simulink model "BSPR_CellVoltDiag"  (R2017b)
settings: Solver=FixedStepDiscrete  StartTime=0.0  StopTime=10.0  FixedStep=0.02  RelTol=1e-3  EnableMultiTasking=on
undefined symbols (not defined in the file): bin2dec, BSPR_bCellVoltAlrmDiag_C, BSPR_CellNplDetVoltThres_C, BSPR_cntCellAvlNum_C, BSPR_cntCellVltRngEnvtCsdr_CW, BSPR_cntCellVoltNplDiag_CW, BSPR_cntCellVoltRngDiag_CW, BSPR_cntModuAvlNum_C, BSPR_cntUCellNplErrThres_C, BSPR_cntUCellNplOkThres_C, BSPR_cntVoltCellMeanSwt_CW, BSPR_cofCurrFltCellRng_C, BSPR_iCellVoltRngCurrHi_C, BSPR_iCellVoltRngCurrLo_C, BSPR_iCurrHopFltDiff_C, BSPR_tBattTempCellVoltRngHi_C, BSPR_tBattTempCellVoltRngLo_C, BSPR_tEnvTCellVoltRngHi_C, BSPR_tEnvTCellVoltRnglo_C, BSPR_tiCellVoltAlrm_C, BSPR_tiCellVoltDiagTask_C, BSPR_tiCellVoltFault_C, BSPR_tiCellVoltFusf_C, BSPR_tiCellVoltWarn_C, BSPR_tiUCellNplErrThres_C, BSPR_tiUCellNplOkThres_C, BSPR_uCellVoltNplDiag_CUR, BSPR_uCellVoltNplDiag_CUR_X, BSPR_uCellVoltRng_CUR_X, BSPR_uCellVoltRng_CUR_Y, BSPR_uCellVoltRngHiFault_CUR, BSPR_uCellVoltRngHiFusf_CUR, BSPR_uCellVoltRngHiWarnAlrm_CUR, BSPR_uCellVoltRngLoFault_CUR, BSPR_uCellVoltRngLoFusf_CUR, BSPR_uCellVoltRngLoWarnAlrm_CUR
libraries: simulink x68, AIWAYS_Powertrain_BMS_lib x9
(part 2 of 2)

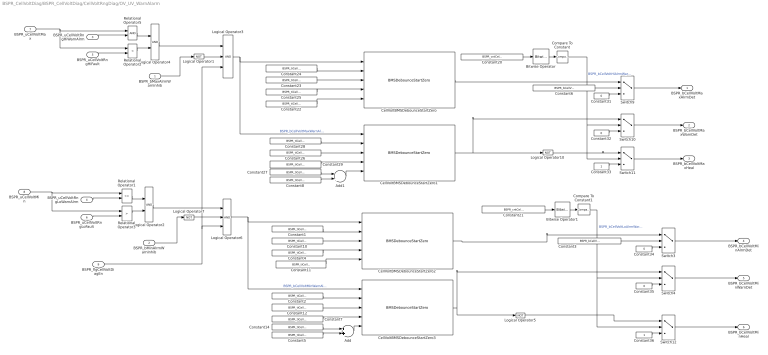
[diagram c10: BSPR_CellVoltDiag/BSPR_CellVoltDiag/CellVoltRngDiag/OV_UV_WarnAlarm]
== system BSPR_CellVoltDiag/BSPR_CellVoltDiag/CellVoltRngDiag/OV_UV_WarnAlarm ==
  BSPR_bMaxAlrmWarnInhib : Inport
  BSPR_bMinAlrmWarnInhib : Inport  Port=2
  BSPR_uCellVoltRngHiWarnAlrm : Inport  Port=3
  BSPR_uCellVoltRngLoWarnAlrm : Inport  Port=4
  BSPR_uCellVoltRngHiFault : Inport  Port=5
  BSPR_uCellVoltRngLoFault : Inport  Port=6
  BSPR_uCellVoltMax : Inport  Port=7
  BSPR_uCellVoltMin : Inport  Port=8
  BSPR_flgCellVoltDiagEn : Inport  Port=9
  Add : Sum
  Add1 : Sum
  Bitwise Operator : simulink/Logic and Bit Operations/Bitwise Operator  logicop=AND  UseBitMask=on  BitMask=bin2dec('00000001')  BitMaskRealWorld=Stored Integer
  Bitwise Operator1 : simulink/Logic and Bit Operations/Bitwise Operator  logicop=AND  UseBitMask=on  BitMask=bin2dec('00000010')  BitMaskRealWorld=Stored Integer
  CellVoltBMSDebounceStartZero{,1..3} (4 alike) : AIWAYS_Powertrain_BMS_lib/Debounce & Delay/BMSDebounceStartZero
  Compare To Constant : simulink/Logic and Bit Operations/Compare To Constant  relop===  const=1  OutDataTypeStr=boolean
  Compare To Constant1 : simulink/Logic and Bit Operations/Compare To Constant  relop===  const=2  OutDataTypeStr=boolean
  Constant1 : Constant  Value=BSPR_tiCellVoltAlrm_C
  Constant{5,8,10..12,14,22..23,26..27} (10 alike) : Constant  Value=BSPR_tiCellVoltDiagTask_C
  Constant{2,4,7,25,28..29} (6 alike) : Constant  Value=BSPR_tiCellVoltWarn_C
  Constant20 : Constant  Value=BSPR_cntCellVoltRngDiag_CW
  Constant21 : Constant  Value=BSPR_cntCellVoltRngDiag_CW
  Constant24 : Constant  Value=BSPR_tiCellVoltAlrm_C
  Constant3 : Constant  Value=BSPR_bCellVoltAlrmDiag_C
  Constant{31..32,34..35} (4 alike) : Constant  Value=0  OutDataTypeStr=boolean
  Constant33 : Constant  OutDataTypeStr=boolean
  Constant36 : Constant  OutDataTypeStr=boolean
  Constant6 : Constant  Value=BSPR_bCellVoltAlrmDiag_C
  Logical Operator{1,5,7,10} (4 alike) : Logic  Operator=NOT  AllPortsSameDT=off  OutDataTypeStr=boolean
  Logical Operator2 : Logic  AllPortsSameDT=off  OutDataTypeStr=boolean
  Logical Operator3 : Logic  Inputs=3  AllPortsSameDT=off  OutDataTypeStr=boolean
  Logical Operator4 : Logic  AllPortsSameDT=off  OutDataTypeStr=boolean
  Logical Operator6 : Logic  Inputs=3  AllPortsSameDT=off  OutDataTypeStr=boolean
  Relational Operator1 : RelationalOperator  Operator=<=  OutDataTypeStr=boolean  RndMeth=Simplest
  Relational Operator2 : RelationalOperator  Operator=<  OutDataTypeStr=boolean  RndMeth=Simplest
  Relational Operator3 : RelationalOperator  Operator=>  OutDataTypeStr=boolean  RndMeth=Simplest
  Relational Operator5 : RelationalOperator  OutDataTypeStr=boolean  RndMeth=Simplest
  Switch{3..4,9..12} (6 alike) : Switch  Criteria=u2 > Threshold
  BSPR_bCellVoltMaxAlrmDet : Outport
  BSPR_bCellVoltMaxWarnDet : Outport  Port=2
  BSPR_bCellVoltMaxHeal : Outport  Port=3
  BSPR_bCellVoltMinAlrmDet : Outport  Port=4
  BSPR_bCellVoltMinWarnDet : Outport  Port=5
  BSPR_bCellVoltMinHeal : Outport  Port=6
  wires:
  BSPR_uCellVoltMax/1 -> Relational Operator2/1, Relational Operator5/1
  BSPR_uCellVoltRngHiWarnAlrm/1 -> Relational Operator5/2
  BSPR_uCellVoltRngLoWarnAlrm/1 -> Relational Operator1/2
  BSPR_uCellVoltMin/1 -> Relational Operator1/1, Relational Operator3/1
  Logical Operator3/1 -> CellVoltBMSDebounceStartZero1/1, CellVoltBMSDebounceStartZero/1  "BSPR_bCellVoltMaxWarnAlrm"
  Logical Operator6/1 -> CellVoltBMSDebounceStartZero3/1, CellVoltBMSDebounceStartZero2/1  "BSPR_bCellVoltMinWarnAlrm"
  BSPR_bMinAlrmWarnInhib/1 -> Logical Operator7/1
  BSPR_uCellVoltRngHiFault/1 -> Relational Operator2/2
  Relational Operator5/1 -> Logical Operator4/1
  Relational Operator2/1 -> Logical Operator4/2
  BSPR_uCellVoltRngLoFault/1 -> Relational Operator3/2
  Relational Operator3/1 -> Logical Operator2/2
  Relational Operator1/1 -> Logical Operator2/1
  BSPR_bMaxAlrmWarnInhib/1 -> Logical Operator1/1
  Compare To Constant/1 -> Switch10/2, Switch11/2  "BSPR_bCellVoltHiAlrmWarnSwt"
  Constant20/1 -> Bitwise Operator/1
  Bitwise Operator/1 -> Compare To Constant/1
  Constant21/1 -> Bitwise Operator1/1
  Bitwise Operator1/1 -> Compare To Constant1/1
  Logical Operator4/1 -> Logical Operator3/1
  Logical Operator2/1 -> Logical Operator6/1
  BSPR_flgCellVoltDiagEn/1 -> Logical Operator3/3, Logical Operator6/3
  Constant22/1 -> CellVoltBMSDebounceStartZero/5
  Constant23/1 -> CellVoltBMSDebounceStartZero/3
  Constant24/1 -> CellVoltBMSDebounceStartZero/2
  Constant25/1 -> CellVoltBMSDebounceStartZero/4
  Constant28/1 -> CellVoltBMSDebounceStartZero1/2
  Constant26/1 -> CellVoltBMSDebounceStartZero1/3
  Constant27/1 -> Add1/1
  Constant29/1 -> CellVoltBMSDebounceStartZero1/4
  CellVoltBMSDebounceStartZero/1 -> Switch9/1
  CellVoltBMSDebounceStartZero1/1 -> Switch10/1, Logical Operator10/1
  Constant31/1 -> Switch9/3
  Constant32/1 -> Switch10/3
  Constant33/1 -> Switch11/3
  Switch9/1 -> BSPR_bCellVoltMaxAlrmDet/1
  Switch10/1 -> BSPR_bCellVoltMaxWarnDet/1
  Switch11/1 -> BSPR_bCellVoltMaxHeal/1
  Logical Operator10/1 -> Switch11/1
  Constant1/1 -> CellVoltBMSDebounceStartZero2/2
  Constant2/1 -> CellVoltBMSDebounceStartZero3/2
  Constant4/1 -> CellVoltBMSDebounceStartZero2/4
  Constant7/1 -> CellVoltBMSDebounceStartZero3/4
  Constant10/1 -> CellVoltBMSDebounceStartZero2/3
  Constant11/1 -> CellVoltBMSDebounceStartZero2/5
  Constant12/1 -> CellVoltBMSDebounceStartZero3/3
  Constant14/1 -> Add/1
  CellVoltBMSDebounceStartZero2/1 -> Switch3/1
  Switch12/1 -> BSPR_bCellVoltMinHeal/1
  Constant36/1 -> Switch12/3
  Compare To Constant1/1 -> Switch12/2, Switch4/2  "BSPR_bCellVoltLoAlrmWarnSwt"
  Switch4/1 -> BSPR_bCellVoltMinWarnDet/1
  Constant34/1 -> Switch3/3
  Switch3/1 -> BSPR_bCellVoltMinAlrmDet/1
  Constant35/1 -> Switch4/3
  CellVoltBMSDebounceStartZero3/1 -> Switch4/1, Logical Operator5/1
  Logical Operator5/1 -> Switch12/1
  Logical Operator1/1 -> Logical Operator3/2
  Logical Operator7/1 -> Logical Operator6/2
  Constant3/1 -> Switch3/2
  Constant5/1 -> Add/2
  Add/1 -> CellVoltBMSDebounceStartZero3/5
  Constant6/1 -> Switch9/2
  Constant8/1 -> Add1/2
  Add1/1 -> CellVoltBMSDebounceStartZero1/5

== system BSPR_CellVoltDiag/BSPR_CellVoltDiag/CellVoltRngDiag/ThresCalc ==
  BSER_rSoh : Inport
  BSPR_tCellTempMax : Inport  Port=2
  BSPR_tCellTempMin : Inport  Port=3
  BSPR_uCellVoltRngHiFault_CUR : Lookup_n-D  LookupTableObject=qdwq  BreakpointsForDimension1=BSPR_uCellVoltRng_CUR_X  BreakpointsForDimension2=BSPR_uCellVoltRng_CUR_Y  Table=BSPR_uCellVoltRngHiFault_CUR  InternalRulePriority=Speed  OutMin=[0]  OutMax=[100]  RndMeth=Simplest  SaturateOnIntegerOverflow=on
  BSPR_uCellVoltRngHiFusf_CUR : Lookup_n-D  LookupTableObject=qdwq  BreakpointsForDimension1=BSPR_uCellVoltRng_CUR_X  BreakpointsForDimension2=BSPR_uCellVoltRng_CUR_Y  Table=BSPR_uCellVoltRngHiFusf_CUR  InternalRulePriority=Speed  OutMin=[0]  OutMax=[100]  RndMeth=Simplest  SaturateOnIntegerOverflow=on
  BSPR_uCellVoltRngHiWarnAlrm_CUR : Lookup_n-D  LookupTableObject=qdwq  BreakpointsForDimension1=BSPR_uCellVoltRng_CUR_X  BreakpointsForDimension2=BSPR_uCellVoltRng_CUR_Y  Table=BSPR_uCellVoltRngHiWarnAlrm_CUR  InternalRulePriority=Speed  OutMin=[0]  OutMax=[100]  RndMeth=Simplest  SaturateOnIntegerOverflow=on
  BSPR_uCellVoltRngLoFault_CUR : Lookup_n-D  LookupTableObject=qdwq  BreakpointsForDimension1=BSPR_uCellVoltRng_CUR_X  BreakpointsForDimension2=BSPR_uCellVoltRng_CUR_Y  Table=BSPR_uCellVoltRngLoFault_CUR  InternalRulePriority=Speed  OutMin=[0]  OutMax=[100]  RndMeth=Simplest  SaturateOnIntegerOverflow=on
  BSPR_uCellVoltRngLoFusf_CUR : Lookup_n-D  LookupTableObject=qdwq  BreakpointsForDimension1=BSPR_uCellVoltRng_CUR_X  BreakpointsForDimension2=BSPR_uCellVoltRng_CUR_Y  Table=BSPR_uCellVoltRngLoFusf_CUR  InternalRulePriority=Speed  OutMin=[0]  OutMax=[100]  RndMeth=Simplest  SaturateOnIntegerOverflow=on
  BSPR_uCellVoltRngLoWarnAlrm_CUR : Lookup_n-D  LookupTableObject=qdwq  BreakpointsForDimension1=BSPR_uCellVoltRng_CUR_X  BreakpointsForDimension2=BSPR_uCellVoltRng_CUR_Y  Table=BSPR_uCellVoltRngLoWarnAlrm_CUR  InternalRulePriority=Speed  OutMin=[0]  OutMax=[100]  RndMeth=Simplest  SaturateOnIntegerOverflow=on
  BSPR_uCellVoltRngHiWarnAlrm : Outport
  BSPR_uCellVoltRngLoWarnAlrm : Outport  Port=2
  BSPR_uCellVoltRngHiFault : Outport  Port=3
  BSPR_uCellVoltRngLoFault : Outport  Port=4
  BSPR_uCellVoltRngHiFusf : Outport  Port=5
  BSPR_uCellVoltRngLoFusf : Outport  Port=6
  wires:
  BSPR_uCellVoltRngHiWarnAlrm_CUR/1 -> BSPR_uCellVoltRngHiWarnAlrm/1  "BSPR_uCellVoltRngHiWarnAlrm"
  BSPR_uCellVoltRngHiFault_CUR/1 -> BSPR_uCellVoltRngHiFault/1  "BSPR_uCellVoltRngHiFault"
  BSPR_uCellVoltRngHiFusf_CUR/1 -> BSPR_uCellVoltRngHiFusf/1  "BSPR_uCellVoltRngHiFusf"
  BSPR_uCellVoltRngLoWarnAlrm_CUR/1 -> BSPR_uCellVoltRngLoWarnAlrm/1  "BSPR_uCellVoltRngLoWarnAlrm"
  BSPR_uCellVoltRngLoFault_CUR/1 -> BSPR_uCellVoltRngLoFault/1  "BSPR_uCellVoltRngLoFault"
  BSPR_uCellVoltRngLoFusf_CUR/1 -> BSPR_uCellVoltRngLoFusf/1  "BSPR_uCellVoltRngLoFusf"
  BSER_rSoh/1 -> BSPR_uCellVoltRngHiFusf_CUR/1, BSPR_uCellVoltRngLoWarnAlrm_CUR/1, BSPR_uCellVoltRngLoFusf_CUR/1, BSPR_uCellVoltRngLoFault_CUR/1, BSPR_uCellVoltRngHiFault_CUR/1, BSPR_uCellVoltRngHiWarnAlrm_CUR/1
  BSPR_tCellTempMax/1 -> BSPR_uCellVoltRngHiFusf_CUR/2, BSPR_uCellVoltRngHiFault_CUR/2, BSPR_uCellVoltRngHiWarnAlrm_CUR/2
  BSPR_tCellTempMin/1 -> BSPR_uCellVoltRngLoWarnAlrm_CUR/2, BSPR_uCellVoltRngLoFusf_CUR/2, BSPR_uCellVoltRngLoFault_CUR/2

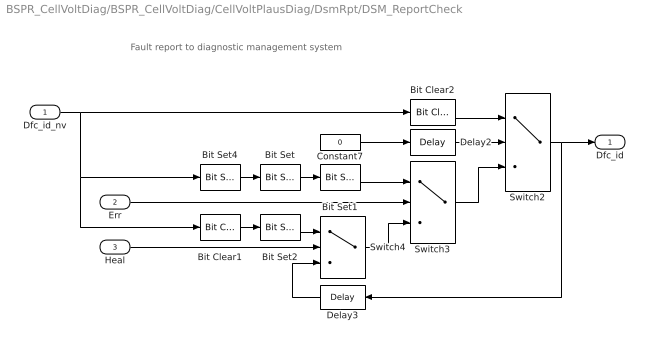
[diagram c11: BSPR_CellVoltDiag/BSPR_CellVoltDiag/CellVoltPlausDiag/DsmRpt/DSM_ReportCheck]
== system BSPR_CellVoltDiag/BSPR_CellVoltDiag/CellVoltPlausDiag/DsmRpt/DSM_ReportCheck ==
  note: Fault report to diagnostic management system
  Dfc_id_nv : Inport  OutDataTypeStr=uint8
  Err : Inport  Port=2
  Heal : Inport  Port=3
  Bit Clear1 : simulink/Logic and Bit Operations/Bit Clear  iBit=4
  Bit Clear2 : simulink/Logic and Bit Operations/Bit Clear  iBit=3
  Bit Set : simulink/Logic and Bit Operations/Bit Set  iBit=4
  Bit Set1 : simulink/Logic and Bit Operations/Bit Set  iBit=3
  Bit Set2 : simulink/Logic and Bit Operations/Bit Set  iBit=3
  Bit Set4 : simulink/Logic and Bit Operations/Bit Set  iBit=7
  Constant7 : Constant  Value=0  OutDataTypeStr=boolean
  Delay2 : Delay  DelayLength=1  InitialCondition=1
  Delay3 : Delay  DelayLength=1  InitialCondition=0
  Switch2 : Switch  Criteria=u2 ~= 0
  Switch3 : Switch  Criteria=u2 ~= 0
  Switch4 : Switch  Criteria=u2 ~= 0
  Dfc_id : Outport  OutDataTypeStr=uint8
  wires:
  Dfc_id_nv/1 -> Bit Clear2/1, Bit Set4/1, Bit Clear1/1
  Bit Set4/1 -> Bit Set/1
  Constant7/1 -> Delay2/1
  Delay2/1 -> Switch2/2
  Switch3/1 -> Switch2/3
  Bit Clear2/1 -> Switch2/1
  Switch2/1 -> Delay3/1, Dfc_id/1
  Bit Set1/1 -> Switch3/1
  Bit Set/1 -> Bit Set1/1
  Switch4/1 -> Switch3/3
  Err/1 -> Switch3/2
  Bit Set2/1 -> Switch4/1
  Bit Clear1/1 -> Bit Set2/1
  Delay3/1 -> Switch4/3
  Heal/1 -> Switch4/2

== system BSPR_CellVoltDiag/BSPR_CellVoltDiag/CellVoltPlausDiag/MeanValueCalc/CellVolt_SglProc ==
  BSPR_uCellVolt_A : Inport
  BSPR_cntCellSerNum : Inport  Port=2
  CompareCalc_CellVolt : Stateflow chart  TreatAsAtomicUnit=on
  Constant1 : Constant  Value=BSPR_cntCellAvlNum_C
  Sum of Elements : Sum  Inputs=+
  SumCalc_CellExtmVolt : Stateflow chart  TreatAsAtomicUnit=on
  Terminator : Terminator
  BSPR_uSumVoltCellTmp : Outport
  BSPR_uSumExtmVoltCell : Outport  Port=2
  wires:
  Sum of Elements/1 -> BSPR_uSumVoltCellTmp/1  "BSPR_uSumVoltCellTmp"
  BSPR_uCellVolt_A/1 -> Sum of Elements/1, CompareCalc_CellVolt/1(BSPR_uCellVolt_A)
  Constant1/1 -> SumCalc_CellExtmVolt/3(BSPR_cntCellAvlNum_C)
  CompareCalc_CellVolt/1(Vol_ASD) -> SumCalc_CellExtmVolt/1(BSPR_uCellExtmVolt_A)
  CompareCalc_CellVolt/2(index) -> Terminator/1
  BSPR_cntCellSerNum/1 -> SumCalc_CellExtmVolt/2(BSPR_cntCellSerNum), CompareCalc_CellVolt/2(BSPR_cntCellSerNum)
  SumCalc_CellExtmVolt/1(BSPR_uSumExtmVoltCell) -> BSPR_uSumExtmVoltCell/1  "BSPR_uSumExtmVoltCell"

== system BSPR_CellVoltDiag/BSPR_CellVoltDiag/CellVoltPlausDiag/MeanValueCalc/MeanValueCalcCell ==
  BSPR_uSumVoltCellTmp : Inport
  BSPR_uSumExtmVoltCell : Inport  Port=2
  BSPR_cntCellSerNum : Inport  Port=3
  Constant4 : Constant  Value=BSPR_cntCellAvlNum_C
  Divide : Product  Inputs=*/  OutDataTypeStr=single
  Gain : Gain  Gain=2  OutDataTypeStr=uint8
  Subtract : Sum  Inputs=+-  AccumDataTypeStr=single
  Subtract1 : Sum  Inputs=+-  OutDataTypeStr=uint8
  BSPR_uVoltCellMean : Outport
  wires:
  BSPR_uSumVoltCellTmp/1 -> Subtract/1
  BSPR_uSumExtmVoltCell/1 -> Subtract/2
  Subtract/1 -> Divide/1
  Divide/1 -> BSPR_uVoltCellMean/1
  Subtract1/1 -> Divide/2
  Constant4/1 -> Gain/1
  Gain/1 -> Subtract1/2
  BSPR_cntCellSerNum/1 -> Subtract1/1

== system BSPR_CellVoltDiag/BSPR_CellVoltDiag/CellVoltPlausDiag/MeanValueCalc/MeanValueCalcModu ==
  BSPR_uSumVoltModuTmp : Inport
  BSPR_uSumExtmVoltModu : Inport  Port=2
  BSPR_cntModuSerNum : Inport  Port=3
  Constant : Constant  Value=12  OutDataTypeStr=uint8
  Constant2 : Constant  Value=BSPR_cntModuAvlNum_C
  Divide : Product  Inputs=*/  OutDataTypeStr=single
  Divide1 : Product  Inputs=*/  OutDataTypeStr=single
  Gain : Gain  Gain=2  OutDataTypeStr=uint8
  Subtract : Sum  Inputs=+-  OutDataTypeStr=single
  Subtract1 : Sum  Inputs=+-  OutDataTypeStr=uint8
  BSPR_uVoltModuMean : Outport
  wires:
  BSPR_cntModuSerNum/1 -> Subtract1/1
  Gain/1 -> Subtract1/2
  Constant2/1 -> Gain/1
  Subtract1/1 -> Divide/2
  Divide1/1 -> BSPR_uVoltModuMean/1
  Subtract/1 -> Divide/1
  BSPR_uSumExtmVoltModu/1 -> Subtract/2
  BSPR_uSumVoltModuTmp/1 -> Subtract/1
  Constant/1 -> Divide1/2
  Divide/1 -> Divide1/1

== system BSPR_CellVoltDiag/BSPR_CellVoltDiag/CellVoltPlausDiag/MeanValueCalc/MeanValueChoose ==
  BSPR_uVoltModuMean : Inport
  BSPR_uVoltCellMean : Inport  Port=2
  BSPR_cntCellSerNum : Inport  Port=3
  Constant3 : Constant  Value=BSPR_cntVoltCellMeanSwt_CW
  Index Vector : MultiPortSwitch  DataPortOrder=Zero-based contiguous  Inputs=2  zeroidx=on  OutDataTypeStr=single
  Product : Product
  BSPR_uCellVoltMeanCoord : Outport
  BSPR_uSumVoltCell : Outport  Port=2
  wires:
  BSPR_uVoltCellMean/1 -> Index Vector/2, Product/1
  Constant3/1 -> Index Vector/1
  Index Vector/1 -> BSPR_uCellVoltMeanCoord/1
  BSPR_uVoltModuMean/1 -> Index Vector/3
  BSPR_cntCellSerNum/1 -> Product/2
  Product/1 -> BSPR_uSumVoltCell/1

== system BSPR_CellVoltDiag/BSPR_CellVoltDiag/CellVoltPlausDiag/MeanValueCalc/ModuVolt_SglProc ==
  BSPR_uMdulVolt_A : Inport
  BSPR_cntModuSerNum : Inport  Port=2
  CompareCalc_ModuVolt : Stateflow chart  TreatAsAtomicUnit=on
  Constant1 : Constant  Value=BSPR_cntModuAvlNum_C
  Sum of Elements : Sum  Inputs=+
  SumCalc_ModuExtmVolt : Stateflow chart  TreatAsAtomicUnit=on
  Terminator : Terminator
  BSPR_uSumVoltModuTmp : Outport
  BSPR_uSumExtmVoltModu : Outport  Port=2
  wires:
  SumCalc_ModuExtmVolt/1(BSPR_uSumExtmVoltModu) -> BSPR_uSumExtmVoltModu/1  "BSPR_uSumExtmVoltModu"
  BSPR_cntModuSerNum/1 -> CompareCalc_ModuVolt/2(BSPR_cntModuSerNum), SumCalc_ModuExtmVolt/2(BSPR_cntModuSerNum)
  CompareCalc_ModuVolt/2(index) -> Terminator/1
  CompareCalc_ModuVolt/1(Vol_ASD) -> SumCalc_ModuExtmVolt/1(BSPR_uModuExtmVolt_A)
  Constant1/1 -> SumCalc_ModuExtmVolt/3(BSPR_cntModuAvlNum_C)
  BSPR_uMdulVolt_A/1 -> Sum of Elements/1, CompareCalc_ModuVolt/1(BSPR_uMdulVolt_A)
  Sum of Elements/1 -> BSPR_uSumVoltModuTmp/1  "BSPR_uSumVoltModuTmp"

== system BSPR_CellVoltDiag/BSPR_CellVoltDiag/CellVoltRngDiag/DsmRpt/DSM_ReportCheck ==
  note: Fault report to diagnostic management system
  Dfc_id_nv : Inport  OutDataTypeStr=uint8
  Err : Inport  Port=2
  Heal : Inport  Port=3
  Bit Clear1 : simulink/Logic and Bit Operations/Bit Clear  iBit=4
  Bit Clear2 : simulink/Logic and Bit Operations/Bit Clear  iBit=3
  Bit Set : simulink/Logic and Bit Operations/Bit Set  iBit=4
  Bit Set1 : simulink/Logic and Bit Operations/Bit Set  iBit=3
  Bit Set2 : simulink/Logic and Bit Operations/Bit Set  iBit=3
  Bit Set4 : simulink/Logic and Bit Operations/Bit Set  iBit=7
  Constant7 : Constant  Value=0  OutDataTypeStr=boolean
  Delay2 : Delay  DelayLength=1  InitialCondition=1
  Delay3 : Delay  DelayLength=1  InitialCondition=0
  Switch2 : Switch  Criteria=u2 ~= 0
  Switch3 : Switch  Criteria=u2 ~= 0
  Switch4 : Switch  Criteria=u2 ~= 0
  Dfc_id : Outport  OutDataTypeStr=uint8
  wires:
  Dfc_id_nv/1 -> Bit Clear2/1, Bit Set4/1, Bit Clear1/1
  Bit Set4/1 -> Bit Set/1
  Constant7/1 -> Delay2/1
  Delay2/1 -> Switch2/2
  Switch3/1 -> Switch2/3
  Bit Clear2/1 -> Switch2/1
  Switch2/1 -> Delay3/1, Dfc_id/1
  Bit Set1/1 -> Switch3/1
  Bit Set/1 -> Bit Set1/1
  Switch4/1 -> Switch3/3
  Err/1 -> Switch3/2
  Bit Set2/1 -> Switch4/1
  Bit Clear1/1 -> Bit Set2/1
  Delay3/1 -> Switch4/3
  Heal/1 -> Switch4/2

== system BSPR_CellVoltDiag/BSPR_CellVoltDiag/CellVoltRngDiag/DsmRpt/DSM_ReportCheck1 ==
  note: Fault report to diagnostic management system
  Dfc_id_nv : Inport  OutDataTypeStr=uint8
  Err : Inport  Port=2
  Heal : Inport  Port=3
  Bit Clear1 : simulink/Logic and Bit Operations/Bit Clear  iBit=4
  Bit Clear2 : simulink/Logic and Bit Operations/Bit Clear  iBit=3
  Bit Set : simulink/Logic and Bit Operations/Bit Set  iBit=4
  Bit Set1 : simulink/Logic and Bit Operations/Bit Set  iBit=3
  Bit Set2 : simulink/Logic and Bit Operations/Bit Set  iBit=3
  Bit Set4 : simulink/Logic and Bit Operations/Bit Set  iBit=7
  Constant7 : Constant  Value=0  OutDataTypeStr=boolean
  Delay2 : Delay  DelayLength=1  InitialCondition=1
  Delay3 : Delay  DelayLength=1  InitialCondition=0
  Switch2 : Switch  Criteria=u2 ~= 0
  Switch3 : Switch  Criteria=u2 ~= 0
  Switch4 : Switch  Criteria=u2 ~= 0
  Dfc_id : Outport  OutDataTypeStr=uint8
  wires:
  Heal/1 -> Switch4/2
  Delay3/1 -> Switch4/3
  Bit Clear1/1 -> Bit Set2/1
  Bit Set2/1 -> Switch4/1
  Err/1 -> Switch3/2
  Switch4/1 -> Switch3/3
  Bit Set/1 -> Bit Set1/1
  Bit Set1/1 -> Switch3/1
  Switch2/1 -> Dfc_id/1, Delay3/1
  Bit Clear2/1 -> Switch2/1
  Switch3/1 -> Switch2/3
  Delay2/1 -> Switch2/2
  Constant7/1 -> Delay2/1
  Bit Set4/1 -> Bit Set/1
  Dfc_id_nv/1 -> Bit Clear1/1, Bit Set4/1, Bit Clear2/1

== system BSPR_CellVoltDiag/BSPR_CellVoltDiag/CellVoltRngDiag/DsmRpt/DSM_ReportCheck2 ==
  note: Fault report to diagnostic management system
  Dfc_id_nv : Inport  OutDataTypeStr=uint8
  Err : Inport  Port=2
  Heal : Inport  Port=3
  Bit Clear1 : simulink/Logic and Bit Operations/Bit Clear  iBit=4
  Bit Clear2 : simulink/Logic and Bit Operations/Bit Clear  iBit=3
  Bit Set : simulink/Logic and Bit Operations/Bit Set  iBit=4
  Bit Set1 : simulink/Logic and Bit Operations/Bit Set  iBit=3
  Bit Set2 : simulink/Logic and Bit Operations/Bit Set  iBit=3
  Bit Set4 : simulink/Logic and Bit Operations/Bit Set  iBit=7
  Constant7 : Constant  Value=0  OutDataTypeStr=boolean
  Delay2 : Delay  DelayLength=1  InitialCondition=1
  Delay3 : Delay  DelayLength=1  InitialCondition=0
  Switch2 : Switch  Criteria=u2 ~= 0
  Switch3 : Switch  Criteria=u2 ~= 0
  Switch4 : Switch  Criteria=u2 ~= 0
  Dfc_id : Outport  OutDataTypeStr=uint8
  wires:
  Dfc_id_nv/1 -> Bit Clear2/1, Bit Set4/1, Bit Clear1/1
  Bit Set4/1 -> Bit Set/1
  Constant7/1 -> Delay2/1
  Delay2/1 -> Switch2/2
  Switch3/1 -> Switch2/3
  Bit Clear2/1 -> Switch2/1
  Switch2/1 -> Delay3/1, Dfc_id/1
  Bit Set1/1 -> Switch3/1
  Bit Set/1 -> Bit Set1/1
  Switch4/1 -> Switch3/3
  Err/1 -> Switch3/2
  Bit Set2/1 -> Switch4/1
  Bit Clear1/1 -> Bit Set2/1
  Delay3/1 -> Switch4/3
  Heal/1 -> Switch4/2

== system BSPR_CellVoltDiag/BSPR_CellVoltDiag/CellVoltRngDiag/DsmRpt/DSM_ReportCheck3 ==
  note: Fault report to diagnostic management system
  Dfc_id_nv : Inport  OutDataTypeStr=uint8
  Err : Inport  Port=2
  Heal : Inport  Port=3
  Bit Clear1 : simulink/Logic and Bit Operations/Bit Clear  iBit=4
  Bit Clear2 : simulink/Logic and Bit Operations/Bit Clear  iBit=3
  Bit Set : simulink/Logic and Bit Operations/Bit Set  iBit=4
  Bit Set1 : simulink/Logic and Bit Operations/Bit Set  iBit=3
  Bit Set2 : simulink/Logic and Bit Operations/Bit Set  iBit=3
  Bit Set4 : simulink/Logic and Bit Operations/Bit Set  iBit=7
  Constant7 : Constant  Value=0  OutDataTypeStr=boolean
  Delay2 : Delay  DelayLength=1  InitialCondition=1
  Delay3 : Delay  DelayLength=1  InitialCondition=0
  Switch2 : Switch  Criteria=u2 ~= 0
  Switch3 : Switch  Criteria=u2 ~= 0
  Switch4 : Switch  Criteria=u2 ~= 0
  Dfc_id : Outport  OutDataTypeStr=uint8
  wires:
  Heal/1 -> Switch4/2
  Delay3/1 -> Switch4/3
  Bit Clear1/1 -> Bit Set2/1
  Bit Set2/1 -> Switch4/1
  Err/1 -> Switch3/2
  Switch4/1 -> Switch3/3
  Bit Set/1 -> Bit Set1/1
  Bit Set1/1 -> Switch3/1
  Switch2/1 -> Dfc_id/1, Delay3/1
  Bit Clear2/1 -> Switch2/1
  Switch3/1 -> Switch2/3
  Delay2/1 -> Switch2/2
  Constant7/1 -> Delay2/1
  Bit Set4/1 -> Bit Set/1
  Dfc_id_nv/1 -> Bit Clear1/1, Bit Set4/1, Bit Clear2/1

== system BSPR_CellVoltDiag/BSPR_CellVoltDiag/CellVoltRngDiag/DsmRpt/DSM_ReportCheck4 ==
  note: Fault report to diagnostic management system
  Dfc_id_nv : Inport  OutDataTypeStr=uint8
  Err : Inport  Port=2
  Heal : Inport  Port=3
  Bit Clear1 : simulink/Logic and Bit Operations/Bit Clear  iBit=4
  Bit Clear2 : simulink/Logic and Bit Operations/Bit Clear  iBit=3
  Bit Set : simulink/Logic and Bit Operations/Bit Set  iBit=4
  Bit Set1 : simulink/Logic and Bit Operations/Bit Set  iBit=3
  Bit Set2 : simulink/Logic and Bit Operations/Bit Set  iBit=3
  Bit Set4 : simulink/Logic and Bit Operations/Bit Set  iBit=7
  Constant7 : Constant  Value=0  OutDataTypeStr=boolean
  Delay2 : Delay  DelayLength=1  InitialCondition=1
  Delay3 : Delay  DelayLength=1  InitialCondition=0
  Switch2 : Switch  Criteria=u2 ~= 0
  Switch3 : Switch  Criteria=u2 ~= 0
  Switch4 : Switch  Criteria=u2 ~= 0
  Dfc_id : Outport  OutDataTypeStr=uint8
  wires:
  Dfc_id_nv/1 -> Bit Clear2/1, Bit Set4/1, Bit Clear1/1
  Bit Set4/1 -> Bit Set/1
  Constant7/1 -> Delay2/1
  Delay2/1 -> Switch2/2
  Switch3/1 -> Switch2/3
  Bit Clear2/1 -> Switch2/1
  Switch2/1 -> Delay3/1, Dfc_id/1
  Bit Set1/1 -> Switch3/1
  Bit Set/1 -> Bit Set1/1
  Switch4/1 -> Switch3/3
  Err/1 -> Switch3/2
  Bit Set2/1 -> Switch4/1
  Bit Clear1/1 -> Bit Set2/1
  Delay3/1 -> Switch4/3
  Heal/1 -> Switch4/2

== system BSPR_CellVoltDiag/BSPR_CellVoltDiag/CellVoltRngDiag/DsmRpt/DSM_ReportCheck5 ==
  note: Fault report to diagnostic management system
  Dfc_id_nv : Inport  OutDataTypeStr=uint8
  Err : Inport  Port=2
  Heal : Inport  Port=3
  Bit Clear1 : simulink/Logic and Bit Operations/Bit Clear  iBit=4
  Bit Clear2 : simulink/Logic and Bit Operations/Bit Clear  iBit=3
  Bit Set : simulink/Logic and Bit Operations/Bit Set  iBit=4
  Bit Set1 : simulink/Logic and Bit Operations/Bit Set  iBit=3
  Bit Set2 : simulink/Logic and Bit Operations/Bit Set  iBit=3
  Bit Set4 : simulink/Logic and Bit Operations/Bit Set  iBit=7
  Constant7 : Constant  Value=0  OutDataTypeStr=boolean
  Delay2 : Delay  DelayLength=1  InitialCondition=1
  Delay3 : Delay  DelayLength=1  InitialCondition=0
  Switch2 : Switch  Criteria=u2 ~= 0
  Switch3 : Switch  Criteria=u2 ~= 0
  Switch4 : Switch  Criteria=u2 ~= 0
  Dfc_id : Outport  OutDataTypeStr=uint8
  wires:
  Heal/1 -> Switch4/2
  Delay3/1 -> Switch4/3
  Bit Clear1/1 -> Bit Set2/1
  Bit Set2/1 -> Switch4/1
  Err/1 -> Switch3/2
  Switch4/1 -> Switch3/3
  Bit Set/1 -> Bit Set1/1
  Bit Set1/1 -> Switch3/1
  Switch2/1 -> Dfc_id/1, Delay3/1
  Bit Clear2/1 -> Switch2/1
  Switch3/1 -> Switch2/3
  Delay2/1 -> Switch2/2
  Constant7/1 -> Delay2/1
  Bit Set4/1 -> Bit Set/1
  Dfc_id_nv/1 -> Bit Clear1/1, Bit Set4/1, Bit Clear2/1

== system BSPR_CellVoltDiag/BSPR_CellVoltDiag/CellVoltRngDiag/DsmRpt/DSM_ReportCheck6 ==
  note: Fault report to diagnostic management system
  Dfc_id_nv : Inport  OutDataTypeStr=uint8
  Err : Inport  Port=2
  Heal : Inport  Port=3
  Bit Clear1 : simulink/Logic and Bit Operations/Bit Clear  iBit=4
  Bit Clear2 : simulink/Logic and Bit Operations/Bit Clear  iBit=3
  Bit Set : simulink/Logic and Bit Operations/Bit Set  iBit=4
  Bit Set1 : simulink/Logic and Bit Operations/Bit Set  iBit=3
  Bit Set2 : simulink/Logic and Bit Operations/Bit Set  iBit=3
  Bit Set4 : simulink/Logic and Bit Operations/Bit Set  iBit=7
  Constant7 : Constant  Value=0  OutDataTypeStr=boolean
  Delay2 : Delay  DelayLength=1  InitialCondition=1
  Delay3 : Delay  DelayLength=1  InitialCondition=0
  Switch2 : Switch  Criteria=u2 ~= 0
  Switch3 : Switch  Criteria=u2 ~= 0
  Switch4 : Switch  Criteria=u2 ~= 0
  Dfc_id : Outport  OutDataTypeStr=uint8
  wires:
  Dfc_id_nv/1 -> Bit Clear2/1, Bit Set4/1, Bit Clear1/1
  Bit Set4/1 -> Bit Set/1
  Constant7/1 -> Delay2/1
  Delay2/1 -> Switch2/2
  Switch3/1 -> Switch2/3
  Bit Clear2/1 -> Switch2/1
  Switch2/1 -> Delay3/1, Dfc_id/1
  Bit Set1/1 -> Switch3/1
  Bit Set/1 -> Bit Set1/1
  Switch4/1 -> Switch3/3
  Err/1 -> Switch3/2
  Bit Set2/1 -> Switch4/1
  Bit Clear1/1 -> Bit Set2/1
  Delay3/1 -> Switch4/3
  Heal/1 -> Switch4/2

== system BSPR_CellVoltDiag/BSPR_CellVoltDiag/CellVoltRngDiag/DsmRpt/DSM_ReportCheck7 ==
  note: Fault report to diagnostic management system
  Dfc_id_nv : Inport  OutDataTypeStr=uint8
  Err : Inport  Port=2
  Heal : Inport  Port=3
  Bit Clear1 : simulink/Logic and Bit Operations/Bit Clear  iBit=4
  Bit Clear2 : simulink/Logic and Bit Operations/Bit Clear  iBit=3
  Bit Set : simulink/Logic and Bit Operations/Bit Set  iBit=4
  Bit Set1 : simulink/Logic and Bit Operations/Bit Set  iBit=3
  Bit Set2 : simulink/Logic and Bit Operations/Bit Set  iBit=3
  Bit Set4 : simulink/Logic and Bit Operations/Bit Set  iBit=7
  Constant7 : Constant  Value=0  OutDataTypeStr=boolean
  Delay2 : Delay  DelayLength=1  InitialCondition=1
  Delay3 : Delay  DelayLength=1  InitialCondition=0
  Switch2 : Switch  Criteria=u2 ~= 0
  Switch3 : Switch  Criteria=u2 ~= 0
  Switch4 : Switch  Criteria=u2 ~= 0
  Dfc_id : Outport  OutDataTypeStr=uint8
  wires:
  Heal/1 -> Switch4/2
  Delay3/1 -> Switch4/3
  Bit Clear1/1 -> Bit Set2/1
  Bit Set2/1 -> Switch4/1
  Err/1 -> Switch3/2
  Switch4/1 -> Switch3/3
  Bit Set/1 -> Bit Set1/1
  Bit Set1/1 -> Switch3/1
  Switch2/1 -> Dfc_id/1, Delay3/1
  Bit Clear2/1 -> Switch2/1
  Switch3/1 -> Switch2/3
  Delay2/1 -> Switch2/2
  Constant7/1 -> Delay2/1
  Bit Set4/1 -> Bit Set/1
  Dfc_id_nv/1 -> Bit Clear1/1, Bit Set4/1, Bit Clear2/1

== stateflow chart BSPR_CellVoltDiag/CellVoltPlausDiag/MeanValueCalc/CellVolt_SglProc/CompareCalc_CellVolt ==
  state Sort
    (default) -> (junction 766) : /*Sort*/
    (junction 768) -> (junction 767) : [i<BSPR_cntCellSerNum]
    (junction 766) -> (junction 768) : {i=0;}
    (junction 767) -> (junction 769) : {index[i]=0; Vol_ASD[i]=0; BSPR_uCellVoltDiag_A[i]=BSPR_uCellVolt_A[i];}
    (junction 769) -> (junction 768) : {i++;}
    (junction 768) -> (junction 770) : {[Vol_ASD,index]=sort(BSPR_uCellVoltDiag_A,BSPR_cntCellSerNum);}
  state [f_Vol_ASD,f_index]=sort(f_MINP_CellVol,num) [function]
    (default) -> (junction 724)
    (junction 726) -> (junction 725) : [f_i<num]
    (junction 724) -> (junction 726) : {f_i=0;temp=0;}
    (junction 725) -> (junction 727) : {f_Vol_ASD[f_i]=f_MINP_CellVol[f_i];}
    (junction 727) -> (junction 726) : {f_i++;}
    (junction 726) -> (junction 732) : {f_i=0;}
    (junction 729) -> (junction 730)
    (junction 730) -> (junction 731) : [f_Vol_ASD[f_j]>temp]
    (junction 732) -> (junction 728) : [f_i<num]
    (junction 728) -> (junction 733) : {temp=0;f_index[f_i]=0;f_j=0;}
    (junction 733) -> (junction 729) : [f_j<num]
    (junction 730) -> (junction 736)
    (junction 731) -> (junction 737) : {temp=f_Vol_ASD[f_j]; f_index[f_i]=f_j;}
    (junction 734) -> (junction 732) : {f_i++;}
    (junction 733) -> (junction 734) : {f_Vol_ASD[f_index[f_i]]=0;}
    (junction 735) -> (junction 733) : {f_j++;}
    (junction 732) -> (junction 739) : {f_i=0;}
    (junction 736) -> (junction 735)
    (junction 737) -> (junction 736)
    (junction 739) -> (junction 738) : [f_i<num]
    (junction 738) -> (junction 740) : {f_Vol_ASD[f_i]=f_MINP_CellVol[f_index[f_i]];}
    (junction 740) -> (junction 739) : {f_i++;}
    (junction 739) -> (junction 741)
  (default) -> Sort
  (junction 792) -> Sort
  (junction 789) -> (junction 792)
  Sort -> (junction 787)
  (junction 787) -> (junction 789)
  data: f_MINP_CellVol function_input single; f_Vol_ASD function_output single; f_index function_output uint8; f_i local uint8; f_j local uint8; temp local uint16; num function_input uint8; BSPR_uCellVolt_A input; BSPR_cntCellSerNum input; i local uint8; Vol_ASD output single; index output uint8; BSPR_uCellVoltDiag_A local single

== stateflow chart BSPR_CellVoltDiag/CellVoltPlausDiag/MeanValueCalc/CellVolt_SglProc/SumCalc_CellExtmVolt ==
  state SumCellExtremeVolt_stt
    (default) -> (junction 10) : % SumCellVolt
    (junction 10) -> (junction 11) : {i=0;BSPR_uSumExtmVoltCell=0;}
    (junction 11) -> (junction 9) : [i<BSPR_cntCellAvlNum_C]
    (junction 9) -> (junction 12) : {BSPR_uSumExtmVoltCell=BSPR_uSumExtmVoltCell+BSPR_uCellExtmVolt_A[i];}
    (junction 12) -> (junction 11) : {i = i + 1;}
    (junction 11) -> (junction 13)
    (junction 13) -> (junction 25) : {i=BSPR_cntCellSerNum-BSPR_cntCellAvlNum_C;}
    (junction 25) -> (junction 20) : [i<BSPR_cntCellSerNum]
    (junction 20) -> (junction 24) : {BSPR_uSumExtmVoltCell = BSPR_uSumExtmVoltCell+BSPR_uCellExtmVolt_A[i];}
    (junction 24) -> (junction 25) : {i = i + 1;}
    (junction 25) -> (junction 27)
  (default) -> SumCellExtremeVolt_stt
  (junction 35) -> SumCellExtremeVolt_stt
  (junction 32) -> (junction 35)
  SumCellExtremeVolt_stt -> (junction 31)
  (junction 31) -> (junction 32)
  data: BSPR_uCellExtmVolt_A input; BSPR_uSumExtmVoltCell output; BSPR_cntCellSerNum input; i local uint8; BSPR_cntCellAvlNum_C input

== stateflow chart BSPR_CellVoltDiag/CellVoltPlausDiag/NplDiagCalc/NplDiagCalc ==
  state DiagUCellProc_stt
    (default) -> (junction 98)
    (junction 98) -> (junction 100)
    (junction 100) -> (junction 102)
    (junction 98) -> (junction 96) : [BSPR_flgCellVoltDiagEn]
    (junction 96) -> (junction 10) : /*Compare */
    (junction 9) -> (junction 23) : [abs(BSPR_uCellVolt_A[i]-BSPR_uCellVoltMeanCoord)<=BSPR_uCellVoltNplDiag_CUR]
    (junction 11) -> (junction 9) : [i<BSPR_cntCellSerNum]
    (junction 10) -> (junction 11) : {i=0;}
    (junction 9) -> (junction 12) : {BSPR_bUCellNplErrStt_A[i]=1;}
    (junction 23) -> (junction 25) : {BSPR_bUCellNplErrStt_A[i]=0;}
    (junction 12) -> (junction 11) : {i = i + 1;}
    (junction 11) -> (junction 13) : /*Debounce*/
    (junction 25) -> (junction 12)
    (junction 48) -> (junction 41) : [BSPR_bUCellNplErrStt_A[i]==1]
    (junction 13) -> (junction 51) : {i=0;}
    (junction 51) -> (junction 48) : [i<BSPR_cntCellSerNum]
    (junction 48) -> (junction 49) : {BSPR_cntUCellNplErrHeal_A[i]=BSPR_cntUCellNplErrHeal_A[i]+1; BSPR_cntUCellNplErrDet_A[i]=0;}
    (junction 41) -> (junction 42) : {BSPR_cntUCellNplErrDet_A[i]=BSPR_cntUCellNplErrDet_A[i]+1; BSPR_cntUCellNplErrHeal_A[i]=0;}
    (junction 49) -> (junction 51) : {i = i + 1;}
    (junction 51) -> (junction 86) : /*Output error result*/
    (junction 42) -> (junction 49)
    (junction 86) -> (junction 64) : {i=0;}
    (junction 55) -> (junction 56) : [BSPR_cntUCellNplErrDet_A[i] > BSPR_cntUCellNplErrThres_C]
    (junction 64) -> (junction 55) : [i<BSPR_cntCellSerNum]
    (junction 55) -> (junction 58) : {BSPR_bUCellNplErrDet_A[i]=0;}
    (junction 56) -> (junction 57) : {BSPR_bUCellNplErrDet_A[i]=1; BSPR_cntUCellNplErrDet_A[i] = BSPR_cntUCellNplErrThres_C;}
    (junction 58) -> (junction 64) : {i = i + 1;}
    (junction 64) -> (junction 84) : /*Output ok result*/
    (junction 57) -> (junction 58)
    (junction 84) -> (junction 69) : {i=0;}
    (junction 67) -> (junction 73) : [BSPR_cntUCellNplErrHeal_A[i] > BSPR_cntUCellNplOkThres_C]
    (junction 69) -> (junction 67) : [i<BSPR_cntCellSerNum]
    (junction 67) -> (junction 70) : {BSPR_bUCellNplErrHeal_A[i]=0;}
    (junction 73) -> (junction 74) : {BSPR_bUCellNplErrHeal_A[i]=1; BSPR_cntUCellNplErrHeal_A[i] = BSPR_cntUCellNplOkThres_C;}
    (junction 70) -> (junction 69) : {i = i + 1;}
    (junction 69) -> (junction 78)
    (junction 74) -> (junction 70)
    (junction 102) -> (junction 78)
  (default) -> DiagUCellProc_stt
  (junction 93) -> DiagUCellProc_stt
  (junction 91) -> (junction 93)
  DiagUCellProc_stt -> (junction 89)
  (junction 89) -> (junction 91)
  data: BSPR_uCellVoltMeanCoord input; BSPR_uCellVolt_A input; BSPR_bUCellNplErrDet_A output; BSPR_uCellVoltNplDiag_CUR input; BSPR_flgCellVoltDiagEn input; i local uint8; BSPR_cntCellSerNum input; BSPR_bUCellNplErrHeal_A output; BSPR_cntUCellNplOkThres_C input; BSPR_cntUCellNplErrThres_C input; BSPR_bUCellNplErrStt_A output; BSPR_cntUCellNplErrDet_A output uint16; BSPR_cntUCellNplErrHeal_A output uint16

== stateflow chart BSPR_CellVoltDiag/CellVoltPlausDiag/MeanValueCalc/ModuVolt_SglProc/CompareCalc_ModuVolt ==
  state Sort
    (default) -> (junction 766) : /*Sort*/
    (junction 768) -> (junction 767) : [i<BSPR_cntModuSerNum]
    (junction 766) -> (junction 768) : {i=0;}
    (junction 767) -> (junction 769) : {index[i]=0; Vol_ASD[i]=0; BSPR_uModuVoltDiag_A[i]=BSPR_uMdulVolt_A[i];}
    (junction 769) -> (junction 768) : {i++;}
    (junction 768) -> (junction 770) : {[Vol_ASD,index]=sort(BSPR_uModuVoltDiag_A,BSPR_cntModuSerNum);}
  state [f_Vol_ASD,f_index]=sort(f_MINP_CellVol,num) [function]
    (default) -> (junction 724)
    (junction 726) -> (junction 725) : [f_i<num]
    (junction 724) -> (junction 726) : {f_i=0;temp=0;}
    (junction 725) -> (junction 727) : {f_Vol_ASD[f_i]=f_MINP_CellVol[f_i];}
    (junction 727) -> (junction 726) : {f_i++;}
    (junction 726) -> (junction 732) : {f_i=0;}
    (junction 729) -> (junction 730)
    (junction 730) -> (junction 731) : [f_Vol_ASD[f_j]>temp]
    (junction 732) -> (junction 728) : [f_i<num]
    (junction 728) -> (junction 733) : {temp=0;f_index[f_i]=0;f_j=0;}
    (junction 733) -> (junction 729) : [f_j<num]
    (junction 730) -> (junction 736)
    (junction 731) -> (junction 737) : {temp=f_Vol_ASD[f_j]; f_index[f_i]=f_j;}
    (junction 734) -> (junction 732) : {f_i++;}
    (junction 733) -> (junction 734) : {f_Vol_ASD[f_index[f_i]]=0;}
    (junction 735) -> (junction 733) : {f_j++;}
    (junction 732) -> (junction 739) : {f_i=0;}
    (junction 736) -> (junction 735)
    (junction 737) -> (junction 736)
    (junction 739) -> (junction 738) : [f_i<num]
    (junction 738) -> (junction 740) : {f_Vol_ASD[f_i]=f_MINP_CellVol[f_index[f_i]];}
    (junction 740) -> (junction 739) : {f_i++;}
    (junction 739) -> (junction 741)
  (default) -> Sort
  (junction 790) -> Sort
  (junction 788) -> (junction 790)
  Sort -> (junction 786)
  (junction 786) -> (junction 788)
  data: f_MINP_CellVol function_input single; f_Vol_ASD function_output single; f_index function_output uint8; f_i local uint8; f_j local uint8; temp local uint16; num function_input uint8; BSPR_uMdulVolt_A input; BSPR_cntModuSerNum input; i local uint8; Vol_ASD output single; index output uint8; BSPR_uModuVoltDiag_A local single

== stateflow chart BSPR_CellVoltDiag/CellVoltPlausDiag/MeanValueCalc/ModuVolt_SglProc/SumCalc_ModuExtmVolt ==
  state SumModuExtremeVolt_stt
    (default) -> (junction 10) : % SumExtmVolt
    (junction 11) -> (junction 9) : [i<BSPR_cntModuAvlNum_C]
    (junction 10) -> (junction 11) : {i=0;BSPR_uSumExtmVoltModu=0;}
    (junction 9) -> (junction 12) : {BSPR_uSumExtmVoltModu=BSPR_uSumExtmVoltModu+BSPR_uModuExtmVolt_A[i];}
    (junction 12) -> (junction 11) : {i = i + 1;}
    (junction 11) -> (junction 13)
    (junction 13) -> (junction 25) : {i=BSPR_cntModuSerNum-BSPR_cntModuAvlNum_C;}
    (junction 25) -> (junction 20) : [i<BSPR_cntModuSerNum]
    (junction 20) -> (junction 24) : {BSPR_uSumExtmVoltModu = BSPR_uSumExtmVoltModu+BSPR_uModuExtmVolt_A[i];}
    (junction 24) -> (junction 25) : {i = i + 1;}
    (junction 25) -> (junction 27)
  (default) -> SumModuExtremeVolt_stt
  (junction 35) -> SumModuExtremeVolt_stt
  (junction 33) -> (junction 35)
  SumModuExtremeVolt_stt -> (junction 31)
  (junction 31) -> (junction 33)
  data: BSPR_uModuExtmVolt_A input; BSPR_uSumExtmVoltModu output; BSPR_cntModuSerNum input; i local uint8; BSPR_cntModuAvlNum_C input
